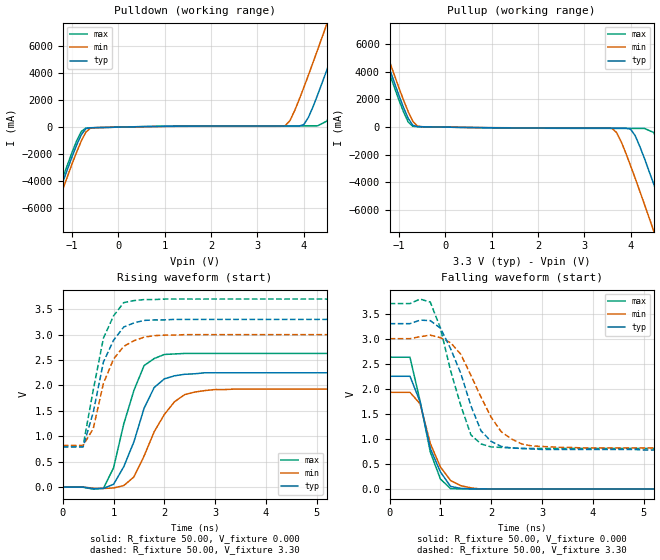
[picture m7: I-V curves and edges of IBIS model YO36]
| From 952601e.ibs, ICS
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|   Model YO36
[Model]   YO36
Model_type   Output
Polarity   Non-Inverting
C_comp   5.50pF   5.00pF   6.00pF
[Temperature Range]   27.00   70.00   0.000
[Voltage Range]   3.30V   3.00V   3.70V
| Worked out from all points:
|   slope of the pulldown table from 0 to 0.495 V, typ, clamps not added: 14.3 ohm
|   slope of the pullup table from 0 to 0.495 V, typ, clamps not added: 20.5 ohm
|   rising waveform, R_fixture 50.00, V_fixture 0.000: 20-80 % time 501ps typ, 600ps min, 449ps max; typ from 0 V to 2.25 V
|   rising waveform, R_fixture 50.00, V_fixture 3.30: 20-80 % time 410ps typ, 411ps min, 382ps max; typ from 0.79 V to 3.3 V
|   falling waveform, R_fixture 50.00, V_fixture 0.000: 20-80 % time 377ps typ, 401ps min, 360ps max; typ from 2.25 V to 0 V
|   falling waveform, R_fixture 50.00, V_fixture 3.30: 20-80 % time 549ps typ, 660ps min, 475ps max; typ from 3.3 V to 0.78 V
[Pulldown]
| voltage   I(typ)   I(min)   I(max)
-3.3V     -24.56A    -25.23A    -24.25A
-1.7V     -8.83A     -9.35A     -8.5A
-1.5V     -6.89A     -7.42A     -6.56A
-900mV    -1.32A     -1.84A     -1.01A
-700mV    -110mA     -360mA     -66.3mA
3.6V      78.43mA    110mA      96.66mA
4V        180mA      2.91A      96.96mA
4.3V      2.38A      5.72A      97.64mA
4.5V      4.23A      7.64A      450mA
4.9V      8.07A      11.53A     3.91A
5.3V      11.98A     15.45A     7.76A
6.6V      24.84A     28.32A     20.57A
[Pullup]
| voltage   I(typ)   I(min)   I(max)
-3.3V     24.68A     25.19A     24.36A
-1.7V     8.94A      9.48A      8.6A
-1.5V     7.01A      7.55A      6.66A
-900mV    1.42A      1.95A      1.1A
-700mV    130mA      420mA      59.96mA
3.6V      -71.58mA   -89.94mA   -90.05mA
4V        -150mA     -2.79A     -91.24mA
4.3V      -2.27A     -5.59A     -92.46mA
4.5V      -4.12A     -7.51A     -390mA
4.9V      -7.96A     -11.4A     -3.8A
5.3V      -11.88A    -15.32A    -7.65A
6.6V      -24.75A    -28.2A     -20.48A
[Ramp]
| variable   typ   min   max
dV/dt_r   1.35/0.43n   1.16/0.59n   1.58/0.36n
dV/dt_f   1.51/0.49n   1.31/0.64n   1.74/0.40n
R_load = 50.00
[Rising Waveform]
R_fixture = 50.00
V_fixture = 0.000
V_fixture_min = 0.000
V_fixture_max = 0.000
| time   V(typ)   V(min)   V(max)
0s        190uV      61.32uV    270uV
800ps     -25.3mV    -26.77mV   -23.68mV
1ns       55.41mV    -16.22mV   380mV
1.2ns     400mV      30.45mV    1.24V
1.4ns     890mV      200mV      1.9V
1.6ns     1.55V      610mV      2.39V
2ns       2.13V      1.43V      2.61V
2.4ns     2.22V      1.82V      2.63V
3ns       2.25V      1.92V      2.63V
10ns      2.25V      1.93V      2.63V
[Rising Waveform]
R_fixture = 50.00
V_fixture = 3.30
V_fixture_min = 3.00
V_fixture_max = 3.70
| time   V(typ)   V(min)   V(max)
0s        790mV      820mV      810mV
400ps     790mV      820mV      810mV
600ps     1.47V      1.15V      1.91V
800ps     2.46V      2.04V      2.93V
1ns       2.89V      2.52V      3.37V
1.2ns     3.15V      2.77V      3.63V
1.4ns     3.23V      2.88V      3.67V
1.6ns     3.28V      2.95V      3.69V
2ns       3.29V      2.99V      3.7V
10ns      3.3V       3V         3.7V
[Falling Waveform]
R_fixture = 50.00
V_fixture = 0.000
V_fixture_min = 0.000
V_fixture_max = 0.000
| time   V(typ)   V(min)   V(max)
0s        2.25V      1.93V      2.63V
400ps     2.25V      1.93V      2.63V
600ps     1.74V      1.7V       1.75V
800ps     810mV      910mV      740mV
1ns       340mV      440mV      200mV
1.2ns     52.66mV    170mV      8.58mV
1.4ns     14.06mV    67.52mV    4.91mV
1.6ns     4.39mV     24.46mV    3.2mV
1.8ns     2.83mV     -170uV     2.08mV
10ns      1.3uV      9.45uV     -2.96uV
[Falling Waveform]
R_fixture = 50.00
V_fixture = 3.30
V_fixture_min = 3.00
V_fixture_max = 3.70
| time   V(typ)   V(min)   V(max)
0s        3.3V       3V         3.7V
800ps     3.36V      3.07V      3.73V
1ns       3.21V      3.02V      3.21V
1.2ns     2.8V       2.92V      2.36V
1.6ns     1.66V      2.27V      1.08V
1.8ns     1.16V      1.83V      900mV
2ns       950mV      1.43V      840mV
2.2ns     850mV      1.14V      830mV
2.8ns     800mV      860mV      810mV
10ns      780mV      820mV      810mV
